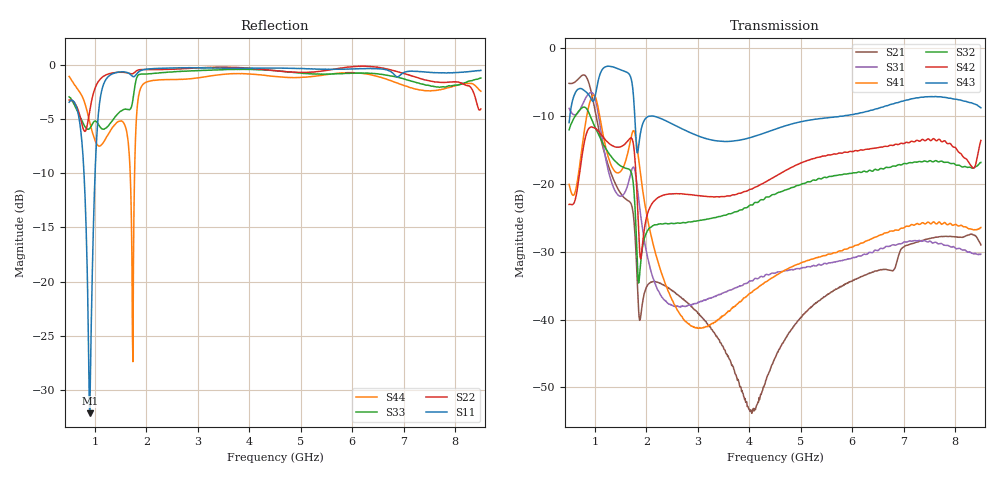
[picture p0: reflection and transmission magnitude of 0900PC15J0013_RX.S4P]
! Pin1 is connected to port3
! Pin2 is connected to port4
!PINS1/2 must be setup as differential ports with: 58-j49ohm differential impedance
! Pin4 is connected to port2, port impedance: 10000ohms
! Pin7 is connected to port1, port impedance: 50ohms
# Hz S RI R 50
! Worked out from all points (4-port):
!   801 points, 500 MHz to 8.5 GHz, reference 50 ohm
!   strongest paths, dB at 500 MHz, 2.5 GHz, 4.5 GHz, 6.5 GHz, 8.5 GHz:
!     S43: -11.0, -11.1, -11.9, -8.9, -8.8
!     S42: -23.0, -21.4, -18.9, -14.7, -13.6
!     S32: -12.0, -25.8, -21.5, -18.0, -16.8
!     S41: -20.1, -37.1, -33.6, -27.7, -26.4
!     S31: -8.9, -37.9, -33.1, -29.8, -30.3
!     S21: -5.2, -35.7, -45.7, -32.8, -29.0
!   lowest |S11| = -32.1 dB at 900 MHz (marker M1), VSWR 1.05, Z = 48.4 + j1.8 ohm
!   |S11| at or under -10 dB: 788.6 MHz to 1.005 GHz (215.9 MHz wide, 24.1 % of centre)
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5e8  0.5011 -0.4453  0.1334 -0.536  0.2467 -0.2602  -0.0112 -0.0969
     0.1331 -0.5358  0.0959 0.6793  0.2439 -0.0521  0.0403 -0.0567
     0.2506 -0.2596  0.2461 -0.0498  -0.6266 0.3327  0.2507 0.1326
     -0.0122 -0.0985  0.0404 -0.058  0.2505 0.1326  -0.3918 0.7894
9e8  -0.0164 0.0186  -0.4786 0.2253  -0.4419 0.1573  0.3439 -0.1936
     -0.4785 0.2252  0.4027 0.46  -0.0852 -0.3124  0.1249 0.2257
     -0.4398 0.1629  -0.0892 -0.3115  0.4544 0.2277  0.4141 -0.1597
     0.3492 -0.1923  0.1238 0.2294  0.4141 -0.1597  0.5351 0.0941
1.14e9  0.7555 0.1506  -0.0128 0.1973  0.1799 0.127  -0.251 0.000787
        -0.0128 0.1973  0.8107 0.3235  -0.1696 -0.1191  0.2239 -0.0244
        0.1778 0.1256  -0.1674 -0.1179  0.2878 -0.4153  0.6352 -0.2817
        -0.2533 -0.00254  0.226 -0.0212  0.6352 -0.2814  -0.3688 -0.2198
2.23e9  -0.1388 -0.9502  0.0177 0.0063  -0.0117 0.0108  -0.0033 -0.0262
        0.0177 0.00623  0.5438 -0.7759  -0.0445 0.0214  0.00789 -0.0793
        -0.0118 0.0114  -0.0452 0.0226  -0.7068 -0.5785  -0.1594 -0.2653
        -0.00325 -0.0262  0.00772 -0.079  -0.1595 -0.265  0.1517 0.8352
4.03e9  -0.9185 -0.2841  0.00207 0.000875  0.000563 0.0197  -0.00968 0.012
        0.00195 0.000928  -0.4189 -0.8634  -0.0232 0.0676  -0.0836 0.0344
        -0.000768 0.0193  -0.027 0.0646  -0.9255 0.2136  -0.124 0.1824
        -0.0102 0.0119  -0.0854 0.033  -0.1241 0.1822  -0.0832 -0.8998
5.97e9  -0.8464 0.4379  0.0096 0.0165  0.0212 0.0174  0.0158 0.0304
        0.0096 0.0165  -0.9763 -0.00827  0.0678 0.0946  0.0217 0.1732
        0.0219 0.0178  0.0697 0.0973  -0.6802 0.607  0.1322 0.2947
        0.0158 0.0303  0.0228 0.1726  0.1321 0.2959  -0.9173 0.0266
8.5e9  -0.1328 0.9303  0.0355 -0.00535  0.0293 -0.00589  0.0479 0.00137
       0.0351 -0.00519  -0.2318 0.5796  0.1435 0.0111  0.1585 0.1386
       0.0297 -0.00678  0.144 0.00771  -0.1547 0.8528  0.3637 0.025
       0.0477 0.00193  0.1557 0.1402  0.3635 0.0263  -0.1047 0.7459
